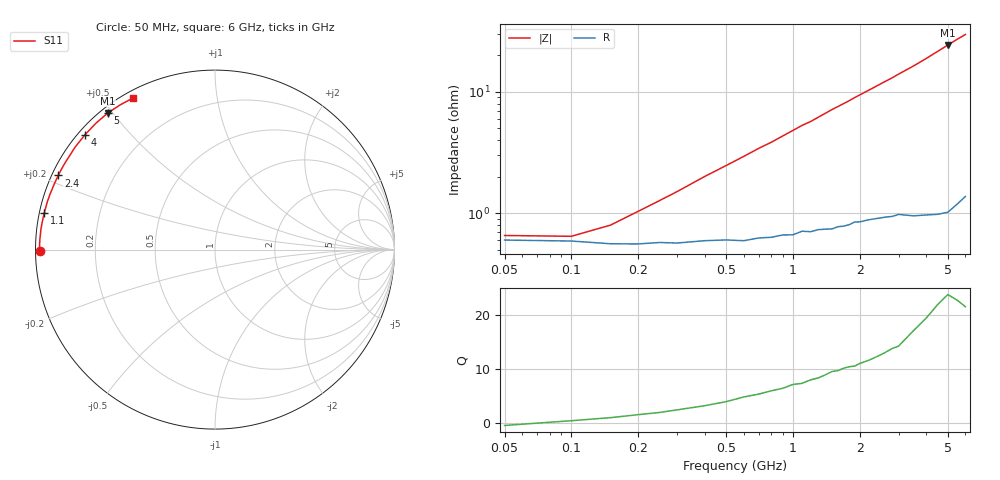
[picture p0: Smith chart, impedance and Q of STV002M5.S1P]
! SIEMENS Discrete & RF Semiconductors
! BA892
! Si PIN Diode in SCD-80
! IF = 2.5 mA
! S-Parameters:  September  1997
# GHz  S  MA  R  50
!  f  S11
! GHz  MAG  ANG
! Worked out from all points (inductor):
!   34 points, 50 MHz to 6 GHz, reference 50 ohm
!   read as one part to ground: L = 764 pH near 400 MHz
!   highest Q = 22.8 at 5 GHz (marker M1), where L = 774 pH
!   S11 on the Smith chart (normalised r, x): 50 MHz: 0.01, -0.01; 1.1 GHz: 0.01, +0.11; 2.4 GHz: 0.02, +0.22; 4 GHz: 0.02, +0.38; 5 GHz: 0.02, +0.49; 6 GHz: 0.03, +0.59
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0.05  0.9762 -179.4
0.1  0.9767 179.4
0.15  0.9778 178.7
0.2  0.9779 178.0
0.3  0.9775 176.8
0.4  0.9766 175.6
0.6  0.9766 173.4
0.7  0.9754 172.3
0.8  0.9751 171.3
1  0.974 169.1
1.1  0.9722 168.0
1.2  0.9726 167.1
1.5  0.9713 163.8
1.6  0.9701 162.8
1.7  0.9699 161.8
1.8  0.9691 160.8
1.9  0.9677 159.7
2  0.9677 158.7
2.4  0.9661 154.7
2.6  0.9656 152.7
2.8  0.9654 150.8
3  0.9644 148.7
3.5  0.9662 143.8
4  0.9667 138.6
4.5  0.9675 133.3
5  0.9676 128.1
5.5  0.964 123.1
6  0.9602 118.5
